(* Logix 5000 AddOnInstructionDefinition export Banner_LCA_Param_v4; software revision 33.00; part 2 of 2 *)
(* tags used below, declared in another part *)
   LCA : Banner_LCA_v4;
   Port_Data : Banner_IOL_Port_v4;
   Port : DINT;
   Local_Control : DINT;
   Command_Being_Processed : BOOL;
   Update_Archive : BOOL;
   Index_Write_Control : DINT;
   Index_Write_Inprocess : INT;
   Inprocess_Index : DINT;
   StatusOut : Banner_LCA_Param_SP_Out_v4[3];
   W_SP_Index : DINT;
(* Banner_LCA_Param_v4, continued *)

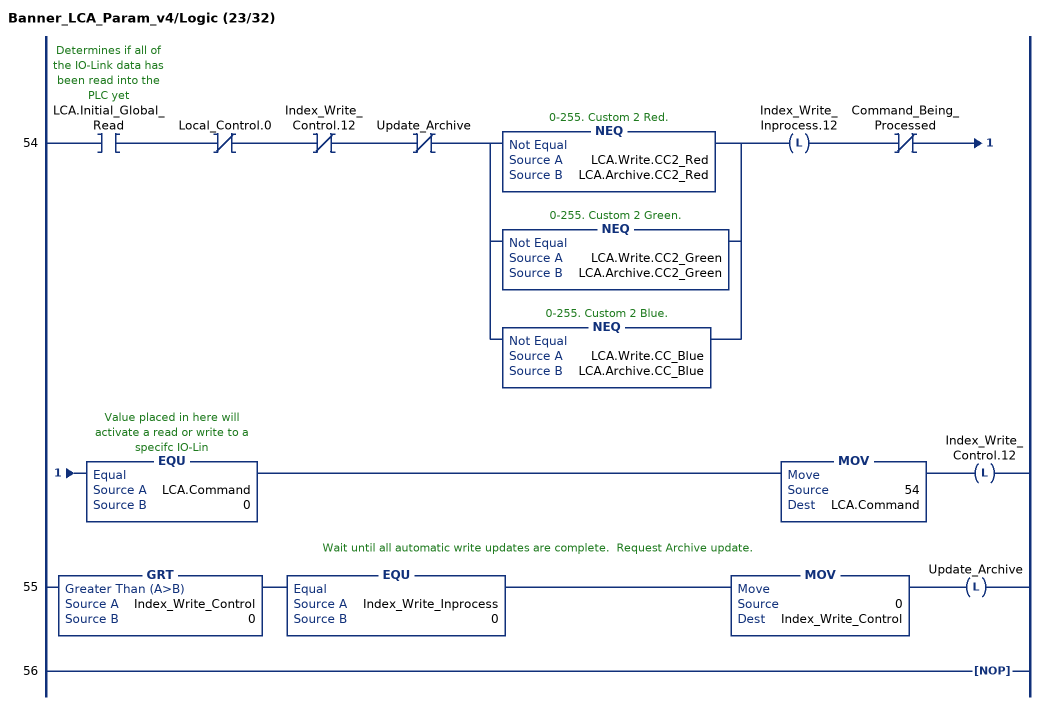
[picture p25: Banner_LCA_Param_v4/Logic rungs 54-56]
   54: XIC(LCA.Initial_Global_Read)XIO(Local_Control.0)XIO(Index_Write_Control.12)XIO(Update_Archive)[NEQ(LCA.Write.CC2_Red,LCA.Archive.CC2_Red) ,NEQ(LCA.Write.CC2_Green,LCA.Archive.CC2_Green) ,NEQ(LCA.Write.CC_Blue,LCA.Archive.CC_Blue) ]OTL(Index_Write_Inprocess.12)XIO(Command_Being_Processed)EQU(LCA.Command,0)MOV(54,LCA.Command)OTL(Index_Write_Control.12);
   // Wait until all automatic write updates are complete.  Request Archive update.
   55: GRT(Index_Write_Control,0)EQU(Index_Write_Inprocess,0)MOV(0,Index_Write_Control)OTL(Update_Archive);
   56: NOP();
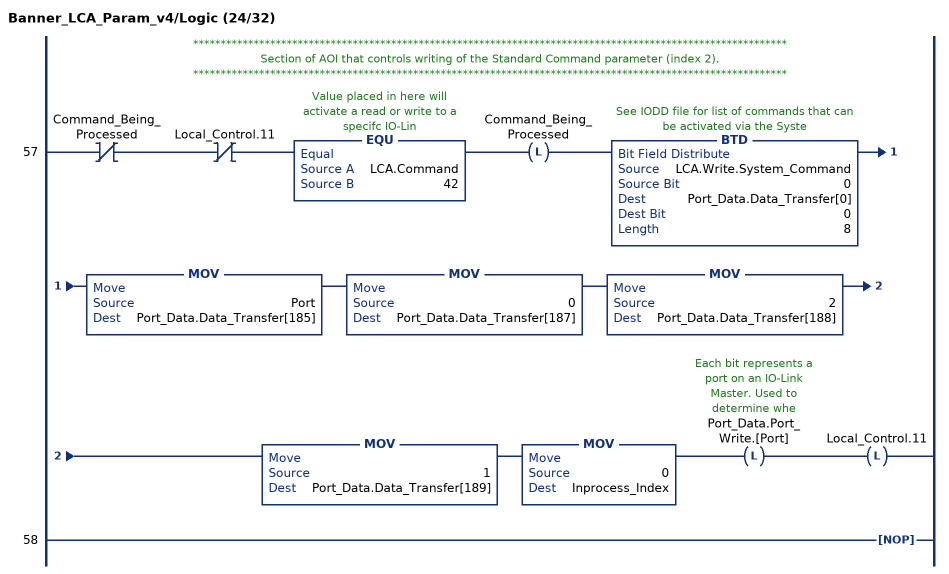
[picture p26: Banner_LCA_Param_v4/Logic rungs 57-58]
   // ************************************************************************************************************
   // Section of AOI that controls writing of the Standard Command parameter (index 2).
   // ************************************************************************************************************
   57: XIO(Command_Being_Processed)XIO(Local_Control.11)EQU(LCA.Command,42)OTL(Command_Being_Processed)BTD(LCA.Write.System_Command,0,Port_Data.Data_Transfer[0],0,8)MOV(Port,Port_Data.Data_Transfer[185])MOV(0,Port_Data.Data_Transfer[187])MOV(2,Port_Data.Data_Transfer[188])MOV(1,Port_Data.Data_Transfer[189])MOV(0,Inprocess_Index)OTL(Port_Data.Port_Write.[Port])OTL(Local_Control.11);
   58: NOP();
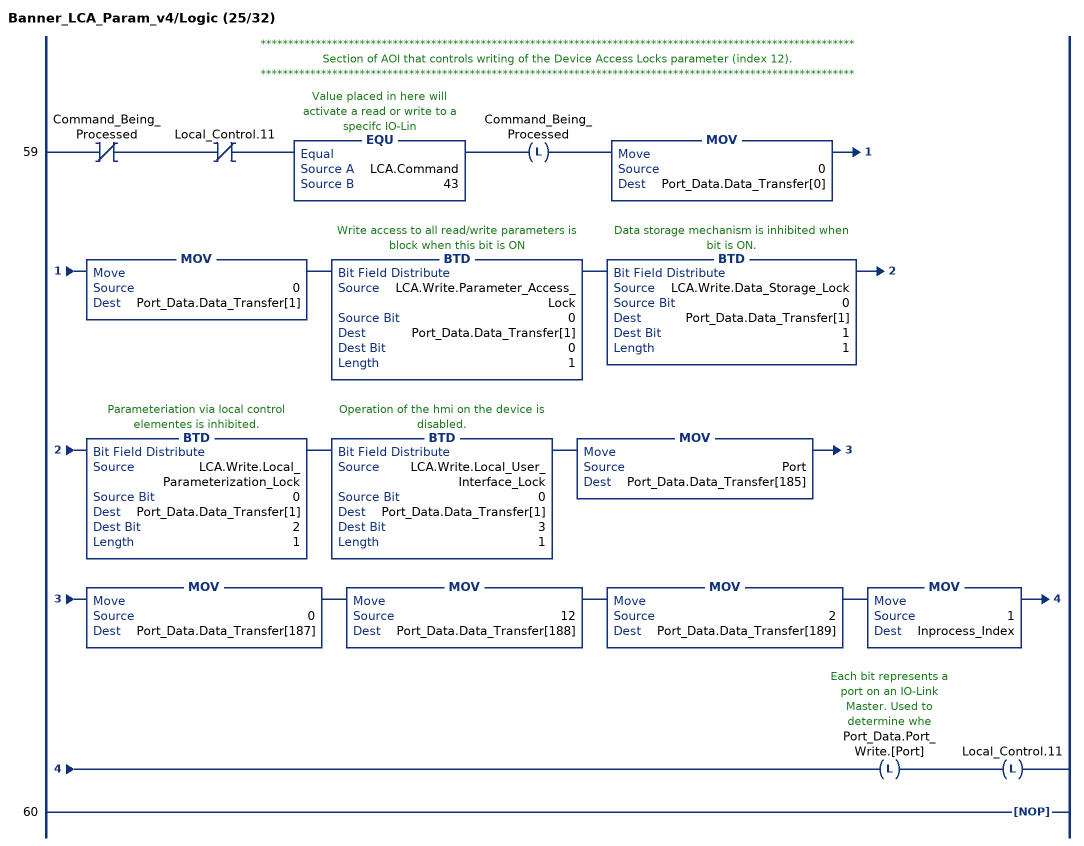
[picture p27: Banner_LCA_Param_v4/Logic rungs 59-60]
   // ************************************************************************************************************
   // Section of AOI that controls writing of the Device Access Locks parameter (index 12).
   // ************************************************************************************************************
   59: XIO(Command_Being_Processed)XIO(Local_Control.11)EQU(LCA.Command,43)OTL(Command_Being_Processed)MOV(0,Port_Data.Data_Transfer[0])MOV(0,Port_Data.Data_Transfer[1])BTD(LCA.Write.Parameter_Access_Lock,0,Port_Data.Data_Transfer[1],0,1)BTD(LCA.Write.Data_Storage_Lock,0,Port_Data.Data_Transfer[1],1,1)BTD(LCA.Write.Local_Parameterization_Lock,0,Port_Data.Data_Transfer[1],2,1)BTD(LCA.Write.Local_User_Interface_Lock,0,Port_Data.Data_Transfer[1],3,1)MOV(Port,Port_Data.Data_Transfer[185])MOV(0,Port_Data.Data_Transfer[187])MOV(12,Port_Data.Data_Transfer[188])MOV(2,Port_Data.Data_Transfer[189])MOV(1,Inprocess_Index)OTL(Port_Data.Port_Write.[Port])OTL(Local_Control.11);
   60: NOP();
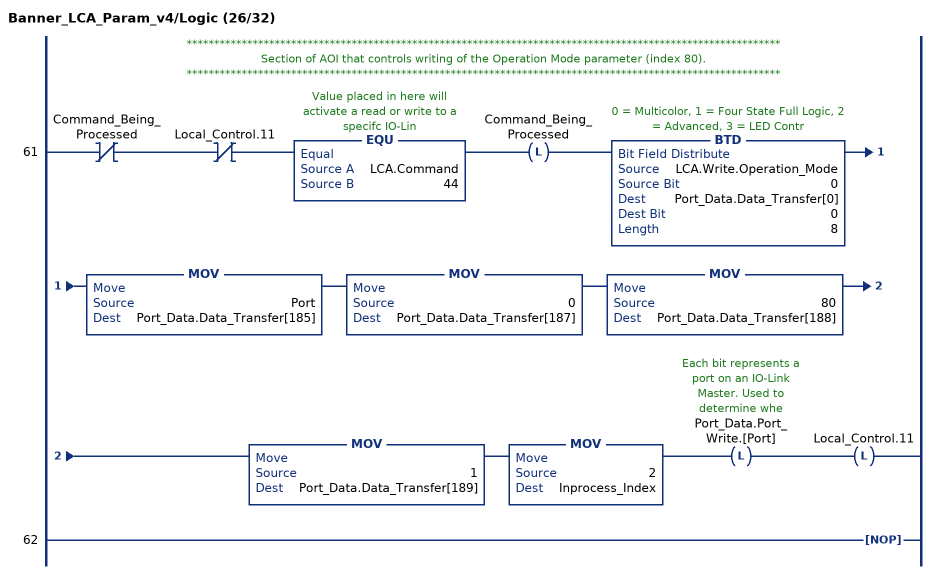
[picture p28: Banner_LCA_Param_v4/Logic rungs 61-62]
   // ************************************************************************************************************
   // Section of AOI that controls writing of the Operation Mode parameter (index 80).
   // ************************************************************************************************************
   61: XIO(Command_Being_Processed)XIO(Local_Control.11)EQU(LCA.Command,44)OTL(Command_Being_Processed)BTD(LCA.Write.Operation_Mode,0,Port_Data.Data_Transfer[0],0,8)MOV(Port,Port_Data.Data_Transfer[185])MOV(0,Port_Data.Data_Transfer[187])MOV(80,Port_Data.Data_Transfer[188])MOV(1,Port_Data.Data_Transfer[189])MOV(2,Inprocess_Index)OTL(Port_Data.Port_Write.[Port])OTL(Local_Control.11);
   62: NOP();
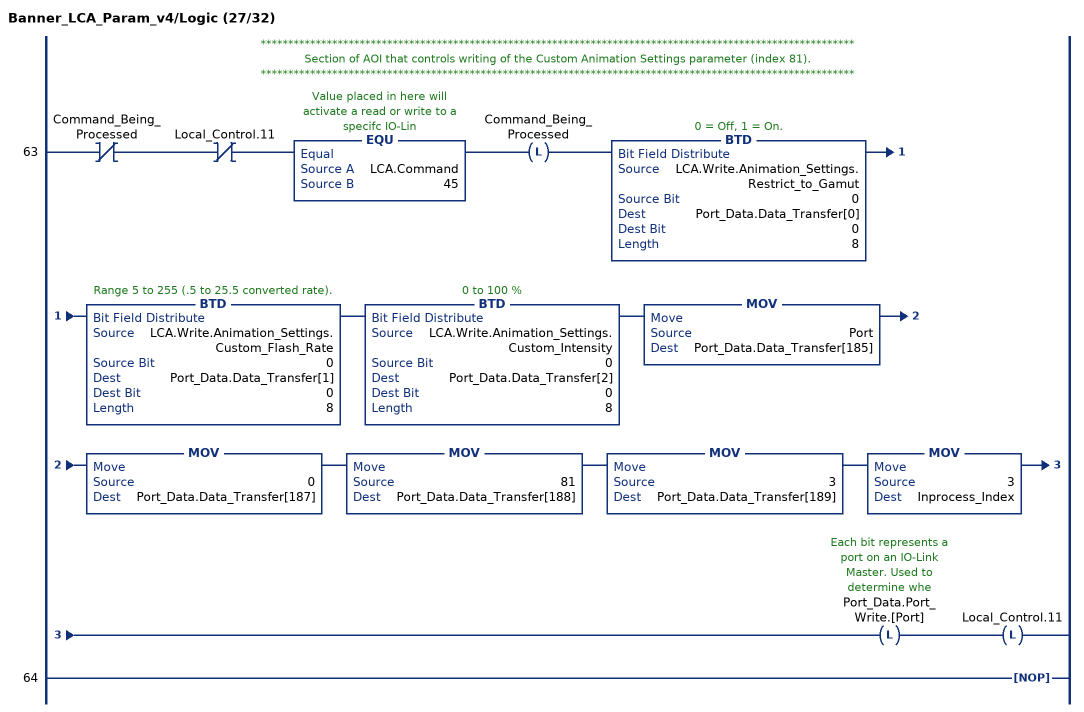
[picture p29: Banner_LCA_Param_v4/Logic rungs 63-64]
   // ************************************************************************************************************
   // Section of AOI that controls writing of the Custom Animation Settings parameter (index 81).
   // ************************************************************************************************************
   63: XIO(Command_Being_Processed)XIO(Local_Control.11)EQU(LCA.Command,45)OTL(Command_Being_Processed)BTD(LCA.Write.Animation_Settings.Restrict_to_Gamut,0,Port_Data.Data_Transfer[0],0,8)BTD(LCA.Write.Animation_Settings.Custom_Flash_Rate,0,Port_Data.Data_Transfer[1],0,8)BTD(LCA.Write.Animation_Settings.Custom_Intensity,0,Port_Data.Data_Transfer[2],0,8)MOV(Port,Port_Data.Data_Transfer[185])MOV(0,Port_Data.Data_Transfer[187])MOV(81,Port_Data.Data_Transfer[188])MOV(3,Port_Data.Data_Transfer[189])MOV(3,Inprocess_Index)OTL(Port_Data.Port_Write.[Port])OTL(Local_Control.11);
   64: NOP();
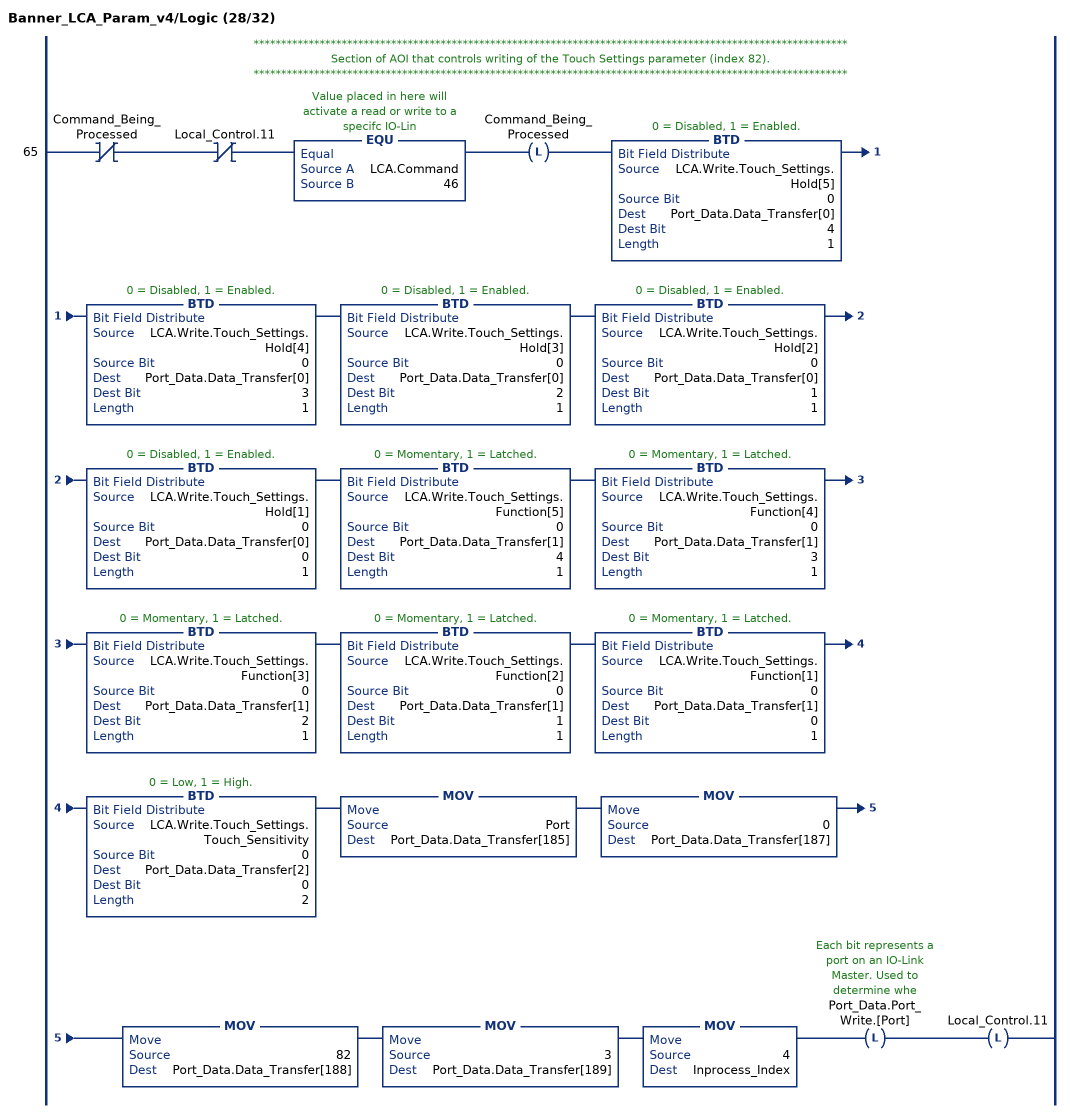
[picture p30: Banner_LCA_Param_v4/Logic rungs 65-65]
   // ************************************************************************************************************
   // Section of AOI that controls writing of the Touch Settings parameter (index 82).
   // ************************************************************************************************************
   65: XIO(Command_Being_Processed)XIO(Local_Control.11)EQU(LCA.Command,46)OTL(Command_Being_Processed)BTD(LCA.Write.Touch_Settings.Hold[5],0,Port_Data.Data_Transfer[0],4,1)BTD(LCA.Write.Touch_Settings.Hold[4],0,Port_Data.Data_Transfer[0],3,1)BTD(LCA.Write.Touch_Settings.Hold[3],0,Port_Data.Data_Transfer[0],2,1)BTD(LCA.Write.Touch_Settings.Hold[2],0,Port_Data.Data_Transfer[0],1,1)BTD(LCA.Write.Touch_Settings.Hold[1],0,Port_Data.Data_Transfer[0],0,1)BTD(LCA.Write.Touch_Settings.Function[5],0,Port_Data.Data_Transfer[1],4,1)BTD(LCA.Write.Touch_Settings.Function[4],0,Port_Data.Data_Transfer[1],3,1)BTD(LCA.Write.Touch_Settings.Function[3],0,Port_Data.Data_Transfer[1],2,1)BTD(LCA.Write.Touch_Settings.Function[2],0,Port_Data.Data_Transfer[1],1,1)BTD(LCA.Write.Touch_Settings.Function[1],0,Port_Data.Data_Transfer[1],0,1)BTD(LCA.Write.Touch_Settings.Touch_Sensitivity,0,Port_Data.Data_Transfer[2],0,2)MOV(Port,Port_Data.Data_Transfer[185])MOV(0,Port_Data.Data_Transfer[187])MOV(82,Port_Data.Data_Transfer[188])MOV(3,Port_Data.Data_Transfer[189])MOV(4,Inprocess_Index)OTL(Port_Data.Port_Write.[Port])OTL(Local_Control.11);
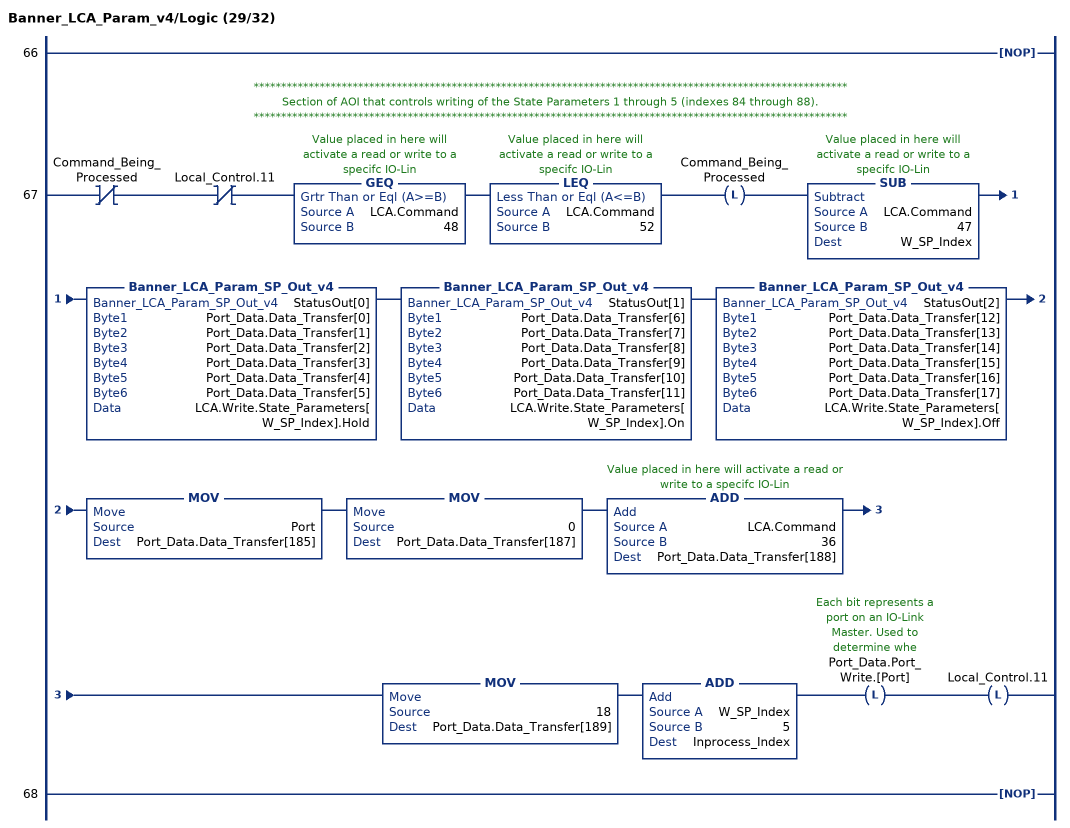
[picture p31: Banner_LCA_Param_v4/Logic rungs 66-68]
   66: NOP();
   // ************************************************************************************************************
   // Section of AOI that controls writing of the State Parameters 1 through 5 (indexes 84 through 88).
   // ************************************************************************************************************
   67: XIO(Command_Being_Processed)XIO(Local_Control.11)GEQ(LCA.Command,48)LEQ(LCA.Command,52)OTL(Command_Being_Processed)SUB(LCA.Command,47,W_SP_Index)Banner_LCA_Param_SP_Out_v4(StatusOut[0],Port_Data.Data_Transfer[0],Port_Data.Data_Transfer[1],Port_Data.Data_Transfer[2],Port_Data.Data_Transfer[3],Port_Data.Data_Transfer[4],Port_Data.Data_Transfer[5],LCA.Write.State_Parameters[W_SP_Index].Hold)Banner_LCA_Param_SP_Out_v4(StatusOut[1],Port_Data.Data_Transfer[6],Port_Data.Data_Transfer[7],Port_Data.Data_Transfer[8],Port_Data.Data_Transfer[9],Port_Data.Data_Transfer[10],Port_Data.Data_Transfer[11],LCA.Write.State_Parameters[W_SP_Index].On)Banner_LCA_Param_SP_Out_v4(StatusOut[2],Port_Data.Data_Transfer[12],Port_Data.Data_Transfer[13],Port_Data.Data_Transfer[14],Port_Data.Data_Transfer[15],Port_Data.Data_Transfer[16],Port_Data.Data_Transfer[17],LCA.Write.State_Parameters[W_SP_Index].Off)MOV(Port,Port_Data.Data_Transfer[185])MOV(0,Port_Data.Data_Transfer[187])ADD(LCA.Command,36,Port_Data.Data_Transfer[188])MOV(18,Port_Data.Data_Transfer[189])ADD(W_SP_Index,5,Inprocess_Index)OTL(Port_Data.Port_Write.[Port])OTL(Local_Control.11);
   68: NOP();
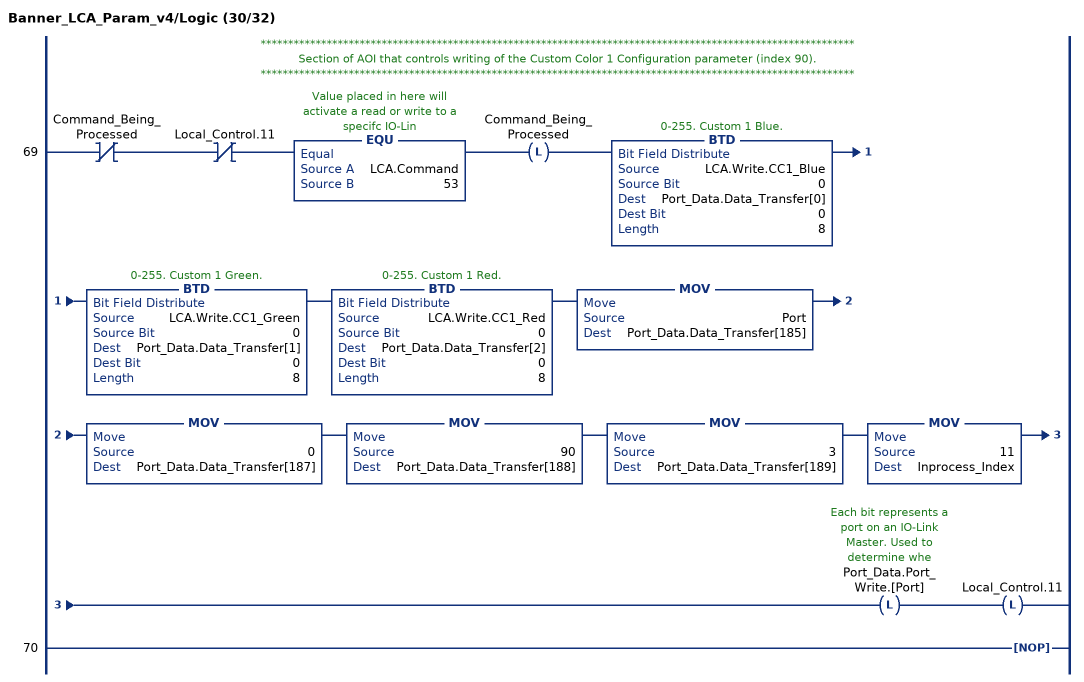
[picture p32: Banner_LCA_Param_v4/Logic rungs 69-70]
   // ************************************************************************************************************
   // Section of AOI that controls writing of the Custom Color 1 Configuration parameter (index 90).
   // ************************************************************************************************************
   69: XIO(Command_Being_Processed)XIO(Local_Control.11)EQU(LCA.Command,53)OTL(Command_Being_Processed)BTD(LCA.Write.CC1_Blue,0,Port_Data.Data_Transfer[0],0,8)BTD(LCA.Write.CC1_Green,0,Port_Data.Data_Transfer[1],0,8)BTD(LCA.Write.CC1_Red,0,Port_Data.Data_Transfer[2],0,8)MOV(Port,Port_Data.Data_Transfer[185])MOV(0,Port_Data.Data_Transfer[187])MOV(90,Port_Data.Data_Transfer[188])MOV(3,Port_Data.Data_Transfer[189])MOV(11,Inprocess_Index)OTL(Port_Data.Port_Write.[Port])OTL(Local_Control.11);
   70: NOP();
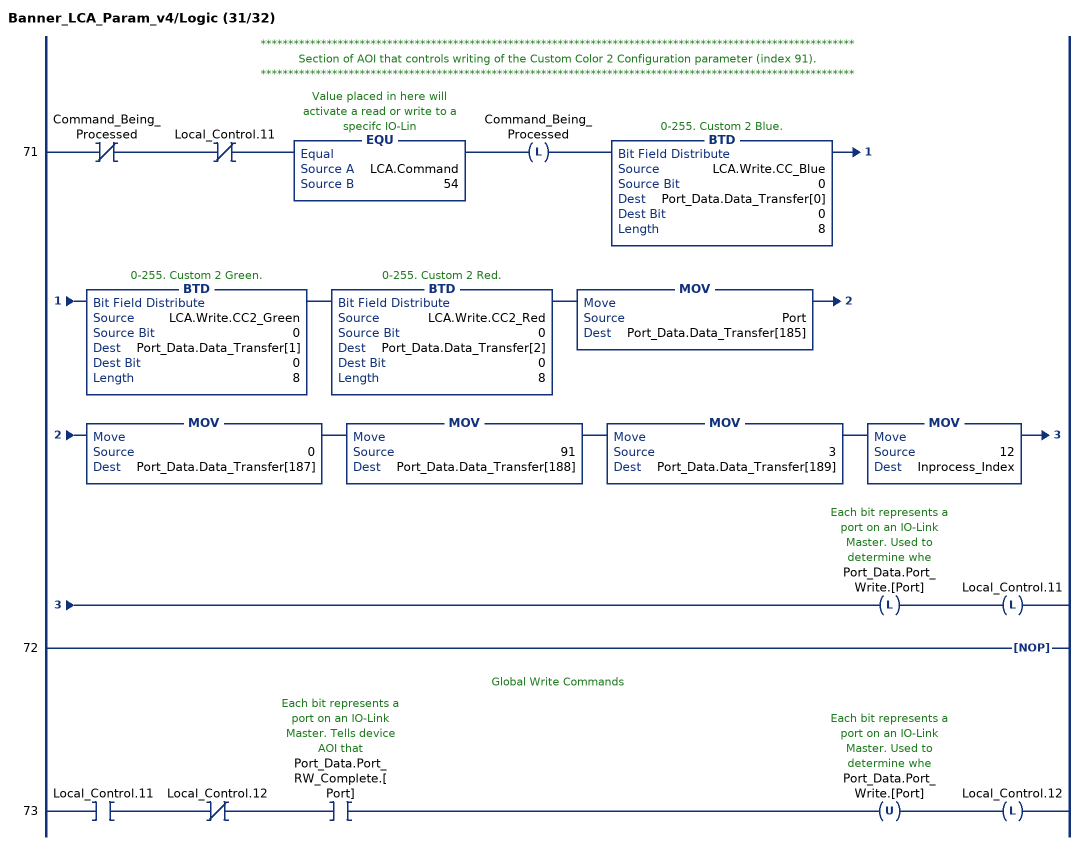
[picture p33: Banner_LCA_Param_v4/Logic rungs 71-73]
   // ************************************************************************************************************
   // Section of AOI that controls writing of the Custom Color 2 Configuration parameter (index 91).
   // ************************************************************************************************************
   71: XIO(Command_Being_Processed)XIO(Local_Control.11)EQU(LCA.Command,54)OTL(Command_Being_Processed)BTD(LCA.Write.CC_Blue,0,Port_Data.Data_Transfer[0],0,8)BTD(LCA.Write.CC2_Green,0,Port_Data.Data_Transfer[1],0,8)BTD(LCA.Write.CC2_Red,0,Port_Data.Data_Transfer[2],0,8)MOV(Port,Port_Data.Data_Transfer[185])MOV(0,Port_Data.Data_Transfer[187])MOV(91,Port_Data.Data_Transfer[188])MOV(3,Port_Data.Data_Transfer[189])MOV(12,Inprocess_Index)OTL(Port_Data.Port_Write.[Port])OTL(Local_Control.11);
   72: NOP();
   // Global Write Commands
   73: XIC(Local_Control.11)XIO(Local_Control.12)XIC(Port_Data.Port_RW_Complete.[Port])OTU(Port_Data.Port_Write.[Port])OTL(Local_Control.12);
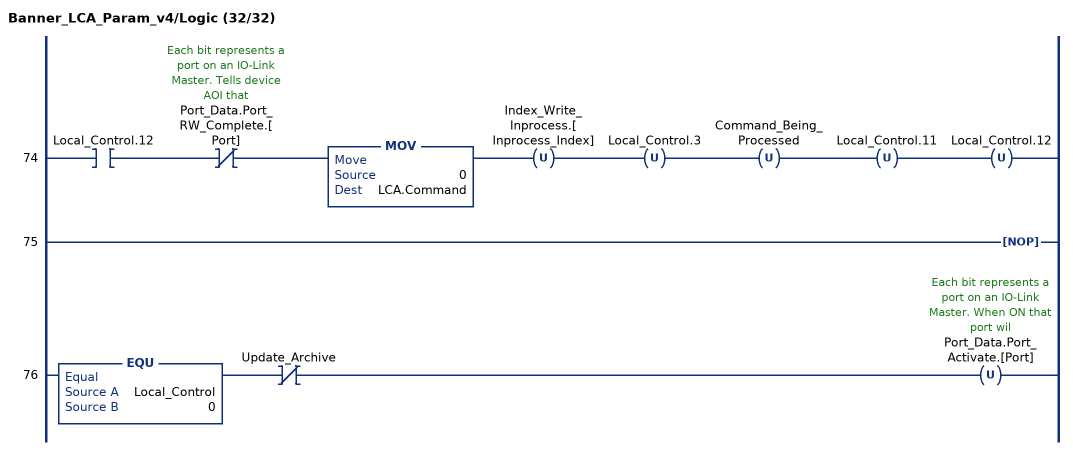
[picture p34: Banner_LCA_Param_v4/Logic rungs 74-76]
   74: XIC(Local_Control.12)XIO(Port_Data.Port_RW_Complete.[Port])MOV(0,LCA.Command)OTU(Index_Write_Inprocess.[Inprocess_Index])OTU(Local_Control.3)OTU(Command_Being_Processed)OTU(Local_Control.11)OTU(Local_Control.12);
   75: NOP();
   76: EQU(Local_Control,0)XIO(Update_Archive)OTU(Port_Data.Port_Activate.[Port]);
END_ROUTINE
END_ADD_ON_INSTRUCTION
